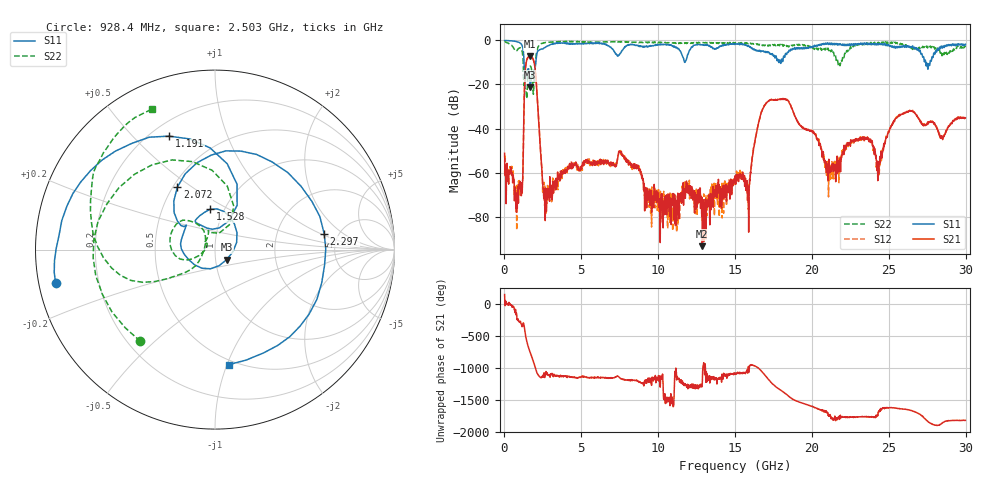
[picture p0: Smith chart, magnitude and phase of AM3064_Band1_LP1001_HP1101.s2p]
# Hz S DB R 50.0
!freq dBS11 angS11 dBS21 angS21 dBS12 angS12 dBS22 angS22
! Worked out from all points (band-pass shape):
!   1600 points, 10 MHz to 29.98 GHz, reference 50 ohm
!   highest |S21| = -7.22 dB at 1.678 GHz (marker M1); lowest = -93.4 dB at 12.87 GHz (marker M2)
!   |S21| within 3 dB of the highest: 1.411 GHz to 1.935 GHz (523.3 MHz wide, 31.3 % of centre)
!   lowest |S11| = -21.4 dB at 1.678 GHz (marker M3), VSWR 1.19, Z = 56.5 - j6.37 ohm
!   |S11| at or under -10 dB: 1.277 GHz to 2.038 GHz (761.2 MHz wide, 45.9 % of centre); 17.94791 GHz to 17.9917 GHz (43.8 MHz wide, 0.244 % of centre); 27.4 GHz to 27.68 GHz (281.2 MHz wide, 1.02 % of centre)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
!   |S22| runs from -26.5 to -0.4 dB; largest |S21 - S12| = 0.0066
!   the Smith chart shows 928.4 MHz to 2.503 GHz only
!   S11 on the Smith chart (normalised r, x): 928.4 MHz: 0.05, -0.10; 1.191 GHz: 0.27, +0.64; 1.528 GHz: 0.86, +0.40; 2.072 GHz: 0.53, +0.44; 2.297 GHz: 3.85, +1.11; 2.503 GHz: 0.46, -1.01
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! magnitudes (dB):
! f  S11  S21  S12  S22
! 10 MHz  -0.1  -51.2  -59.4  -0.4
! 928.4 MHz  -0.8  -66.7  -65.6  -3.6
! 1.191 GHz  -3.3  -63.2  -61.9  -7.1
! 1.528 GHz  -12.9  -7.8  -7.7  -15.3
! 1.678 GHz  -21.4  -7.2  -7.2  -11.7
! 2.072 GHz  -7.8  -19.4  -19.3  -6.0
! 2.297 GHz  -4.2  -43.8  -44.4  -1.8
! 2.503 GHz  -3.8  -66.7  -67.0  -1.3
! 5.015 GHz  -1.3  -58.4  -57.8  -0.7
! 7.582 GHz  -5.5  -51.1  -51.9  -0.5
! 10 GHz  -2.0  -69.4  -74.9  -1.0
! 12.87 GHz  -2.0  -93.4  -79.4  -1.0
! 15 GHz  -1.7  -61.4  -64.3  -1.4
! 15.85 GHz  -2.4  -66.2  -68.3  -1.5
! 16.56 GHz  -4.9  -36.6  -36.3  -2.2
! 17.22 GHz  -5.6  -27.4  -27.5  -2.1
! 19.99 GHz  -3.3  -41.1  -41.4  -3.1
! 21.19 GHz  -1.9  -57.6  -58.0  -4.4
! 23.18 GHz  -1.2  -44.2  -45.4  -2.0
! 24.34 GHz  -2.0  -60.6  -59.5  -1.2
! 25 GHz  -1.9  -41.6  -41.7  -1.0
! 29.98 GHz  -1.8  -35.2  -35.3  -3.1
